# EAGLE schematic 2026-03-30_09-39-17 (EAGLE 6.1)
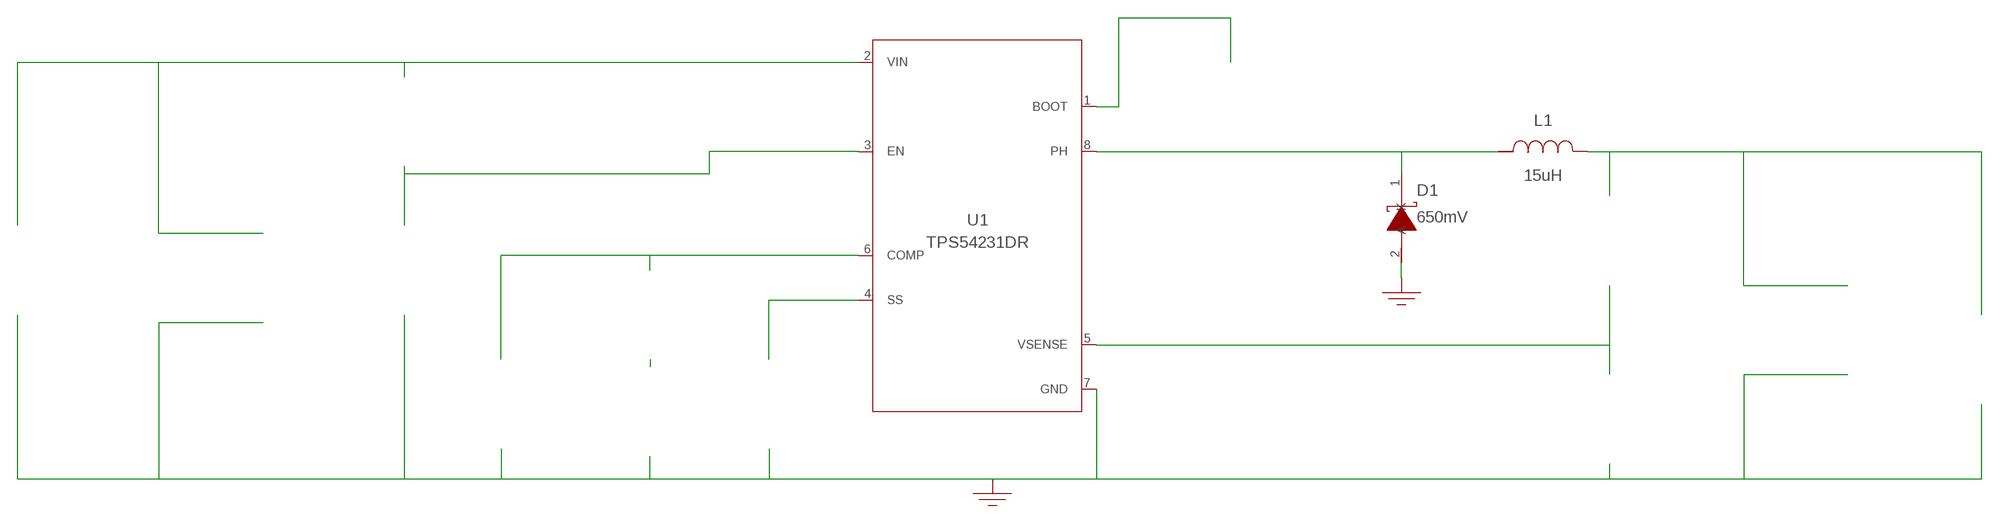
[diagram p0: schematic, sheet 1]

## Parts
CBOOT  100nF  08053C104KAT2A08053C104KAT2A  [0805]  (not placed on a sheet)
CCOMP  1nF  CL21C102JBCNFNCCL21C102JBCNFNC  [0805]  (not placed on a sheet)
CCOMP2  10pF  CC0805JRNPO9BN100CC0805JRNPO9BN100  [0805]  (not placed on a sheet)
CIN  10uF  C3225X7R1H106M250ACC3225X7R1H106M250AC  [1210]  (not placed on a sheet)
CIN_2  10uF  C3225X7R1H106M250ACC3225X7R1H106M250AC  [1210]  (not placed on a sheet)
COUT  47uF  GRM32ER61C476KE15LGRM32ER61C476KE15L  [1210_280]  (not placed on a sheet)
COUT_2  47uF  GRM32ER61C476KE15LGRM32ER61C476KE15L  [1210_280]  (not placed on a sheet)
CSS  8.2nF  12063A822JAT2A12063A822JAT2A  [1206]  (not placed on a sheet)
D1  650mV  FSV360FPFSV360FP  [SOD-123HE]
GND  WB_GND  WB_GNDWB_GND  [WB_GND]
GND2  WB_GND  WB_GNDWB_GND  [WB_GND]
IOUT  WB_CURRENT_LOAD  WB_CURRENT_LOADWB_CURRENT_LOAD  [WB_CURRENT_LOAD]  (not placed on a sheet)
L1  15uH  DR1040-150-RDR1040-150-R  [DR1040]
RCOMP  40.2k  ERJ-6ENF4022VERJ-6ENF4022V  [0805]  (not placed on a sheet)
RENB  15.8k  CRCW080515K8FKEACRCW080515K8FKEA  [0805]  (not placed on a sheet)
RENT  169k  ERJ-6ENF1693VERJ-6ENF1693V  [0805]  (not placed on a sheet)
RFBB  1.96k  ERJ-6ENF1961VERJ-6ENF1961V  [0805]  (not placed on a sheet)
RFBT  10.2k  CRCW080510K2FKEACRCW080510K2FKEA  [0805]  (not placed on a sheet)
U1  TPS54231DR  TPS54231DRTPS54231DR  [D0008A]
VIN  WB_BATTERY  WB_BATTERYWB_BATTERY  [WB_BATTERY]  (not placed on a sheet)
Unconnected: CBOOT.1 CBOOT.2 CCOMP2.1 CCOMP2.2 CCOMP.1 CCOMP.2 CIN.1 CIN.2 CIN_2.1 CIN_2.2 COUT.1 COUT.2 COUT_2.1 COUT_2.2 CSS.1 CSS.2 D1.1(K) D1.2(A) GND2.1 GND.1 IOUT.1(+) IOUT.2(-) L1.1 L1.2 RCOMP.1 RCOMP.2 RENB.1 RENB.2 RENT.1 RENT.2 RFBB.1 RFBB.2 RFBT.1 RFBT.2 U1.1(BOOT) U1.2(VIN) U1.3(EN) U1.4(SS) U1.5(VSENSE) U1.6(COMP) U1.7(GND) U1.8(PH) VIN.1(+) VIN.2(-)

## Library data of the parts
CBOOT = AcceleratedDesigns_Lib:08053C104KAT2A; Manufacturer_Part_Number: 08053C104KAT2A; Vendor: AVX
CCOMP = AcceleratedDesigns_Lib:CL21C102JBCNFNC; Manufacturer_Part_Number: CL21C102JBCNFNC; Vendor: Samsung Electro-Mechanics
CCOMP2 = AcceleratedDesigns_Lib:CC0805JRNPO9BN100; Manufacturer_Part_Number: CC0805JRNPO9BN100; Vendor: Yageo America
CIN CIN_2 = AcceleratedDesigns_Lib:C3225X7R1H106M250AC; Manufacturer_Part_Number: C3225X7R1H106M250AC; Vendor: TDK
COUT COUT_2 = AcceleratedDesigns_Lib:GRM32ER61C476KE15L; Manufacturer_Part_Number: GRM32ER61C476KE15L; Vendor: MuRata
CSS = AcceleratedDesigns_Lib:12063A822JAT2A; Manufacturer_Part_Number: 12063A822JAT2A; Vendor: AVX
D1 = AcceleratedDesigns_Lib:FSV360FP; Manufacturer_Part_Number: FSV360FP; Vendor: Fairchild Semiconductor
GND GND2 = AcceleratedDesigns_Lib:WB_GND; Manufacturer_Part_Number: WB_GND
IOUT = AcceleratedDesigns_Lib:WB_CURRENT_LOAD; Manufacturer_Part_Number: WB_CURRENT_LOAD
L1 = AcceleratedDesigns_Lib:DR1040-150-R; Manufacturer_Part_Number: DR1040-150-R; Vendor: Coiltronics
RCOMP = AcceleratedDesigns_Lib:ERJ-6ENF4022V; Manufacturer_Part_Number: ERJ-6ENF4022V; Vendor: Panasonic
RENB = AcceleratedDesigns_Lib:CRCW080515K8FKEA; Manufacturer_Part_Number: CRCW080515K8FKEA; Vendor: Vishay-Dale
RENT = AcceleratedDesigns_Lib:ERJ-6ENF1693V; Manufacturer_Part_Number: ERJ-6ENF1693V; Vendor: Panasonic
RFBB = AcceleratedDesigns_Lib:ERJ-6ENF1961V; Manufacturer_Part_Number: ERJ-6ENF1961V; Vendor: Panasonic
RFBT = AcceleratedDesigns_Lib:CRCW080510K2FKEA; Manufacturer_Part_Number: CRCW080510K2FKEA; Vendor: Vishay-Dale
U1 = AcceleratedDesigns_Lib:TPS54231DR; Manufacturer_Part_Number: TPS54231DR; Vendor: Texas Instruments
VIN = AcceleratedDesigns_Lib:WB_BATTERY; Manufacturer_Part_Number: WB_BATTERY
